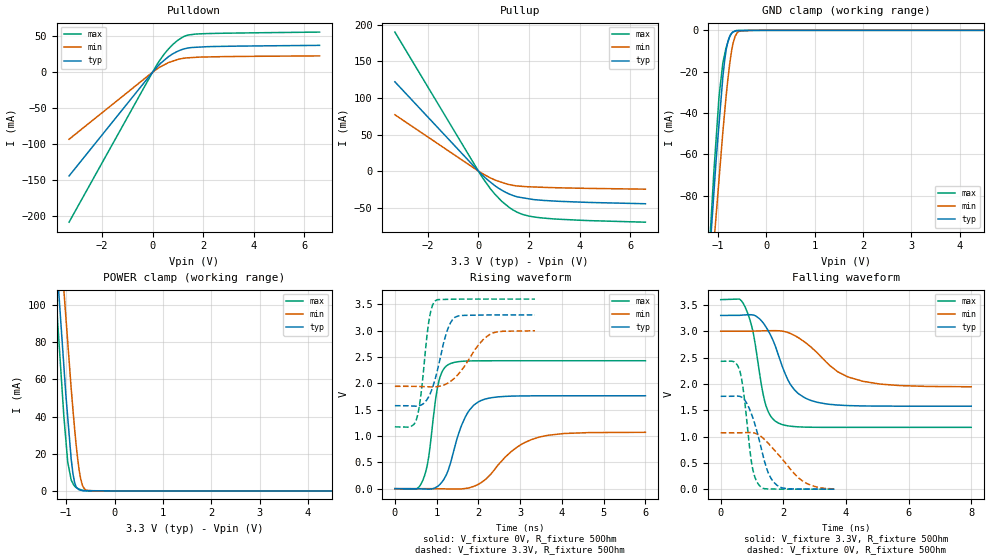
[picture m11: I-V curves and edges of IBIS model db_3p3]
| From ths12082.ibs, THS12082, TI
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|   db_3p3 Model
[Model]   db_3p3
Model_type   I/O
Polarity   Non-Inverting
Enable   Active-High
Vinl = 0.6
Vinh = 2
Vmeas = 1.65
Vref = 1.65
Cref = 30pF
Rref = 50
|   typ   min   max
|   (nom PVT)   (fast PVT)   (slow PVT)
C_comp   1.867e-12   1.852e-12   1.910e-12
|ON state : BUFFER OUTPUT TURNED HIGH
|C_comp   1.978e-12   1.956e-12   2.046e-12
|OFF state: BUFFER IN HIGH IMPEDANCE
|C_comp   1.756e-12   1.747e-12   1.775e-12
| Where nom  PVT is Nominal Process, 3.3V, 27C
|   Fast PVT is Strong Process,  3.6V, -55C
|   Slow PVT is Weak Process,   3V, 125C
[Voltage Range]   3.3   3   3.6
|Ambient Temperature   25   125   -55
|Junction Temperature
[Temperature Range]   27   125   -55
[Pullup Reference]   3.3   3   3.6
[Pulldown Reference]   0   0   0
[Power Clamp Reference]   3.3   3   3.6
[GND Clamp Reference]   0   0   0
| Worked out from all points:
|   slope of the pulldown table from 0 to 0.495 V, typ, clamps not added: 28 ohm
|   slope of the pullup table from 0 to 0.495 V, typ, clamps not added: 31.6 ohm
|   GND clamp passes 1 mA (typ) near -0.70 V on its own axis
|   POWER clamp passes 1 mA (typ) near -0.75 V on its own axis
|   falling waveform, V_fixture 3.3V, R_fixture 50Ohm: 20-80 % time 745ps typ, 1.29ns min, 430ps max; typ from 3.3 V to 1.58 V
|   rising waveform, V_fixture 0V, R_fixture 50Ohm: 20-80 % time 444ps typ, 842ps min, 243ps max; typ from 0 V to 1.76 V
|   rising waveform, V_fixture 3.3V, R_fixture 50Ohm: 20-80 % time 332ps typ, 569ps min, 200ps max; typ from 1.58 V to 3.3 V
|   falling waveform, V_fixture 0V, R_fixture 50Ohm: 20-80 % time 500ps typ, 938ps min, 283ps max; typ from 1.76 V to 0 V
[Pulldown]
|   Voltage   I(typ)   I(min)   I(max)
-3.3V     -144.5mA   -93.38mA   -208.8mA
154.8mV   6.391mA    3.9mA      9.471mA
421.2mV   15.49mA    9.556mA    23.4mA
630mV     21.64mA    13.42mA    32.38mA
1.008V    29.35mA    17.89mA    44.7mA
1.35V     33.32mA    19.96mA    51.22mA
1.804V    34.88mA    20.94mA    53.31mA
6.6V      37.38mA    22.72mA    55.87mA
[GND Clamp]
|   Voltage   I(typ)   I(min)   I(max)
-3.3V     -990.2mA   -935.5mA   -1.082A
-1.224V   -127.2mA   -148.9mA   -125.1mA
-1.084V   -79.04mA   -103.8mA   -68.83mA
-1.059V   -70.63mA   -96.18mA   -60.32mA
-1.033V   -61.71mA   -88.62mA   -51.43mA
-975.6mV  -45.2mA    -72mA      -31.92mA
-896.4mV  -22.48mA   -49.05mA   -15.68mA
-831.6mV  -9.862mA   -32.53mA   -8.589mA
-720mV    -1.591mA   -10.49mA   -1.576mA
-615.6mV  -167.9uA   -1.775mA   -85.91uA
-285mV    -77.23uA   -357.5nA   -40.77nA
6.6V      0A         0A         0A
[Pullup]
|   Voltage   I(typ)   I(min)   I(max)
-3.3V     122.1mA    77.06mA    190.1mA
172.8mV   -6.011mA   -3.66mA    -9.533mA
633.6mV   -19.54mA   -11.88mA   -30.88mA
939.6mV   -26.48mA   -15.57mA   -41.89mA
1.246V    -31.78mA   -18.71mA   -50.45mA
1.512V    -35mA      -20.31mA   -55.96mA
1.75V     -36.55mA   -20.97mA   -59.35mA
2.473V    -39.84mA   -22.12mA   -63.99mA
4.162V    -42.64mA   -23.56mA   -67.49mA
6.6V      -44.7mA    -24.77mA   -69.93mA
[POWER Clamp]
|   Voltage   I(typ)   I(min)   I(max)
-3.3V     1.048A     1.053A     1.062A
-1.218V   131.8mA    172.4mA    107.8mA
-1.175V   114.7mA    156.1mA    90.17mA
-1.035V   62.14mA    103.3mA    36.03mA
-968.4mV  39.53mA    80.07mA    15.51mA
-897.6mV  17.4mA     55.4mA     5.995mA
-861.3mV  9.463mA    44.04mA    4.061mA
-792mV    2.053mA    24.24mA    1.753mA
-726mV    538.4uA    10.19mA    947.2uA
-630mV    157.1uA    1.35mA     156.4uA
-402mV    99.97uA    2.66uA     279.7nA
6.6V      0A         0A         0A
[Ramp]
R_load = 50
|   typ   min   max
dV/dt_r   1.05823/4.43197e-10   0.64203/8.405e-10   1.45735/2.41303e-10
dV/dt_f   1.03447/7.39003e-10   0.633076/1.27256e-09   1.45578/4.28385e-10
[Falling Waveform]
V_fixture = 3.3V
V_fixture_min = 3V
V_fixture_max = 3.6V
R_fixture = 50Ohm
|   Time   V(typ)   V(min)   V(max)
0s        3.3V       3V         3.6V
780ps     3.31V      3V         3.459V
1.038ns   3.309V     3.001V     2.969V
1.43ns    3.095V     3.008V     1.614V
1.838ns   2.551V     3.009V     1.257V
2.356ns   1.885V     2.92V      1.188V
3.058ns   1.654V     2.604V     1.175V
3.738ns   1.598V     2.229V     1.174V
4.528ns   1.581V     2.05V      1.174V
7.998ns   1.576V     1.945V     1.174V
[Rising Waveform]
V_fixture = 0V
V_fixture_min = 0V
V_fixture_max = 0V
R_fixture = 50Ohm
|   Time   V(typ)   V(min)   V(max)
0s        1.442nV    2.279nV    1.191nV
668ps     -5.146mV   243.6uV    156.1mV
810ps     -9.379mV   -33.84uV   605.1mV
1.05ns    60.32mV    -1.879mV   2.029V
1.282ns   362.9mV    -4.928mV   2.357V
1.692ns   1.37V      3.955mV    2.422V
2.064ns   1.674V     113.5mV    2.428V
2.778ns   1.756V     699.2mV    2.429V
3.45ns    1.763V     977.7mV    2.429V
5.998ns   1.764V     1.07V      2.429V
[Rising Waveform]
V_fixture = 3.3V
V_fixture_min = 3V
V_fixture_max = 3.6V
R_fixture = 50Ohm
|   Time   V(typ)   V(min)   V(max)
0s        1.576V     1.943V     1.174V
376ps     1.571V     1.944V     1.176V
518ps     1.567V     1.942V     1.32V
624ps     1.586V     1.939V     1.788V
814ps     1.752V     1.933V     3.179V
958ps     2.065V     1.934V     3.561V
1.252ns   3V         1.997V     3.595V
1.44ns    3.255V     2.108V     3.598V
2.272ns   3.298V     2.928V     3.6V
3.354ns   3.3V       2.998V     3.6V
[Falling Waveform]
V_fixture = 0V
V_fixture_min = 0V
V_fixture_max = 0V
R_fixture = 50Ohm
|   Time   V(typ)   V(min)   V(max)
0s        1.764V     1.07V      2.429V
428ps     1.766V     1.07V      2.42V
612ps     1.762V     1.071V     2.241V
736ps     1.714V     1.073V     1.816V
990ps     1.414V     1.074V     486.2mV
1.228ns   934.9mV    1.026V     73.48mV
1.52ns    307.6mV    870mV      4.549mV
1.796ns   74.33mV    687.2mV    1.772mV
2.602ns   2.318mV    159.5mV    233uV
3.654ns   328.4uV    3.643mV    133.1uV
